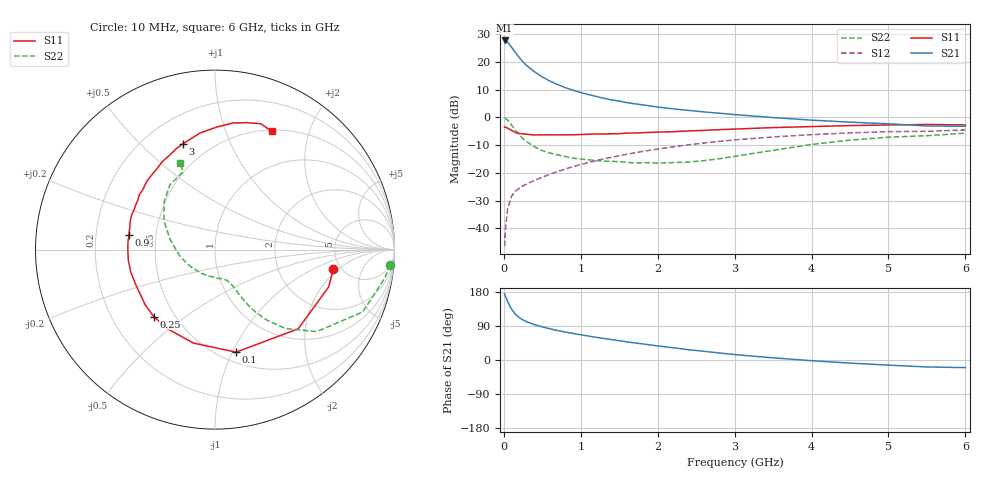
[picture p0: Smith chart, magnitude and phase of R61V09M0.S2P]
! SIEMENS Small Signal Semiconductors
! BFR193
! Si NPN RF Bipolar Junction Transistor in SOT23
! VCE = 1 V  IC = 9 mA
! Common Emitter S-Parameters:  May  1996
# GHz  S  MA  R  50
!  f  S11  S21  S12  S22
! GHz  MAG  ANG  MAG  ANG  MAG  ANG  MAG  ANG
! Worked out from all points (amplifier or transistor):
!   36 points, 10 MHz to 6 GHz, reference 50 ohm
!   highest |S21| = 27.7 dB at 10 MHz (marker M1)
!   |S21| within 3 dB of that: start of sweep to 114.6 MHz
!   unconditionally stable (mu >= 1): 720.1 MHz to 2.195 GHz
!   at 250 MHz: K = 0.62, MSG = 22.3 dB, |S12| = -24.6 dB
!   at 1.4 GHz: K = 1.05, MAG = 8.9 dB, |S12| = -14.4 dB
!   at 6 GHz: K = 0.98, MSG = 0.7 dB, |S12| = -4.5 dB
!   S11 on the Smith chart (normalised r, x): 10 MHz: 4.33, -1.71; 100 MHz: 0.60, -1.03; 250 MHz: 0.38, -0.38; 900 MHz: 0.35, +0.07; 3 GHz: 0.36, +0.68; 6 GHz: 0.52, +1.46
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0.01  0.6688 -9.4  24.28 174.7  0.0048 84.7  0.9788 -4.9
0.02  0.6665 -18.2  24.03 168.9  0.0096 80.5  0.9596 -9.5
0.05  0.6399 -43.6  22.62 153.7  0.023 71.5  0.893 -22.9
0.1  0.5833 -78.4  18.36 134.4  0.0381 60.2  0.7278 -38.9
0.15  0.5346 -103.0  14.64 120.7  0.0468 53.4  0.5886 -48.3
0.2  0.5142 -120.2  11.98 112.0  0.053 51.7  0.485 -53.8
0.25  0.5058 -132.5  9.926 105.5  0.0586 51.3  0.413 -57.1
0.3  0.4957 -141.8  8.507 100.6  0.0637 51.8  0.3646 -59.0
0.4  0.4829 -156.4  6.602 93.3  0.0736 53.4  0.2952 -61.3
0.5  0.4857 -165.3  5.339 87.3  0.0836 55.3  0.2522 -62.8
0.6  0.4864 -173.0  4.5 82.3  0.0948 56.9  0.2283 -63.7
0.7  0.4854 -179.4  3.903 77.6  0.1058 58.0  0.2111 -65.0
0.9  0.4867 170.3  3.085 70.0  0.1299 59.1  0.1842 -68.7
1.1  0.4975 161.9  2.575 63.2  0.1541 59.1  0.1727 -74.0
1.3  0.5022 154.1  2.213 56.7  0.1792 58.2  0.1632 -79.7
1.6  0.5211 144.0  1.842 47.8  0.2167 56.1  0.1552 -91.8
2.2  0.5523 126.6  1.424 32.3  0.2948 49.8  0.1537 -122.0
3  0.6152 107.1  1.123 14.3  0.3938 38.3  0.1987 -169.1
3.5  0.6549 97.3  0.992 5.7  0.4445 30.5  0.2556 167.5
4.5  0.7129 81.8  0.821 -8.2  0.5262 15.5  0.3894 136.7
5.5  0.7463 70.0  0.7 -18.4  0.5614 0.8  0.4688 112.2
6  0.731 64.4  0.693 -20.1  0.5953 -3.6  0.5187 111.9
